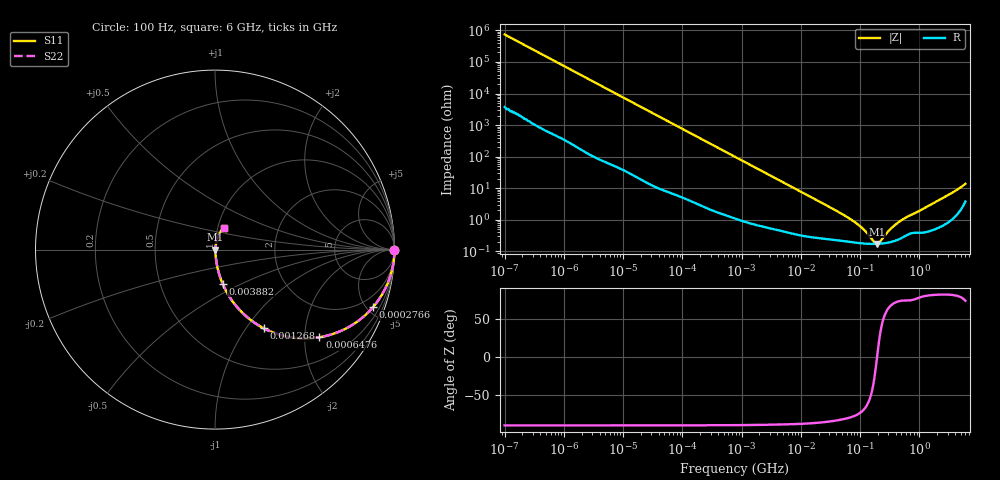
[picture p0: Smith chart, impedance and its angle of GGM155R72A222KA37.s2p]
!Murata Part Number: GGM155R72A222KA37
!These Parameters are Measured in Series Mode Connection
!Data Generated on Jun 19, 2026
!  o--ll--o
!Port1  Port2
!  o------o
!Operation Temp=25[degC], DC Bias Voltage=0[V]
!Freq. Start=100[Hz] Stop=6[GHz] 401[Steps]
# Hz S RI R 50
!Freq.(Hz) S11(Real) S11(Imag) S21(Real) S21(Imag) S12(Real) S12(Imag) S22(Real) S22(Imag)
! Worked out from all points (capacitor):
!   401 points, 100 Hz to 6 GHz, reference 50 ohm
!   read as one part in series: C = 2.14 nF near 109 Hz
!   lowest |Z| = 174 mohm at 190.9 MHz (marker M1)
!   series resonance near 193.5 MHz, so ESL is about 320 pH
!   S11 on the Smith chart (normalised r, x): 100 Hz: open; 276.6 kHz: 1.04, -5.50; 647.6 kHz: 1.02, -2.36; 1.268 MHz: 1.02, -1.21; 3.882 MHz: 1.01, -0.40; 6 GHz: 1.08, +0.27
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100  1 -0.000135  7e-07 0.000135  7e-07 0.000135  1 -0.000135
2008  1 -0.00268  1.88e-05 0.00268  1.88e-05 0.00268  1 -0.00268
40335  0.9969 -0.0532  0.00312 0.0532  0.00312 0.0532  0.9969 -0.0532
112960  0.9773 -0.1454  0.0227 0.1454  0.0227 0.1454  0.9773 -0.1454
276587  0.8814 -0.3193  0.1186 0.3193  0.1186 0.3193  0.8814 -0.3193
413847  0.7705 -0.4161  0.2295 0.4161  0.2295 0.4161  0.7705 -0.4161
647581  0.5813 -0.4881  0.4187 0.4881  0.4187 0.4881  0.5813 -0.4881
774597  0.4939 -0.4944  0.5061 0.4944  0.5061 0.4944  0.4939 -0.4944
1267578  0.2708 -0.4377  0.7292 0.4377  0.7292 0.4377  0.2708 -0.4377
2074311  0.1251 -0.3224  0.8749 0.3224  0.8749 0.3224  0.1251 -0.3224
3882480  0.0424 -0.1898  0.9576 0.1898  0.9576 0.1898  0.0424 -0.1898
1.555665e7  0.00528 -0.0498  0.9947 0.0498  0.9947 0.0498  0.00528 -0.0498
7.797396e7  0.002 -0.00876  0.998 0.00876  0.998 0.00876  0.002 -0.00876
1.115611e8  0.00181 -0.00493  0.9982 0.00493  0.9982 0.00493  0.00181 -0.00493
1.669249e8  0.00173 -0.00127  0.9983 0.00127  0.9983 0.00127  0.00173 -0.00127
1.909225e8  0.00173 -0.000114  0.9983 0.000114  0.9983 0.000114  0.00173 -0.000114
2.183701e8  0.00175 0.00105  0.9982 -0.00105  0.9982 -0.00105  0.00175 0.00105
3.124326e8  0.00194 0.00429  0.9981 -0.00429  0.9981 -0.00429  0.00194 0.00429
4.087225e8  0.00228 0.00702  0.9977 -0.00702  0.9977 -0.00702  0.00228 0.00702
5.59173e8  0.00307 0.0106  0.9969 -0.0106  0.9969 -0.0106  0.00307 0.0106
2.34314e9  0.00813 0.0447  0.9919 -0.0447  0.9919 -0.0447  0.00813 0.0447
6e9  0.052 0.1215  0.948 -0.1215  0.948 -0.1215  0.052 0.1215
